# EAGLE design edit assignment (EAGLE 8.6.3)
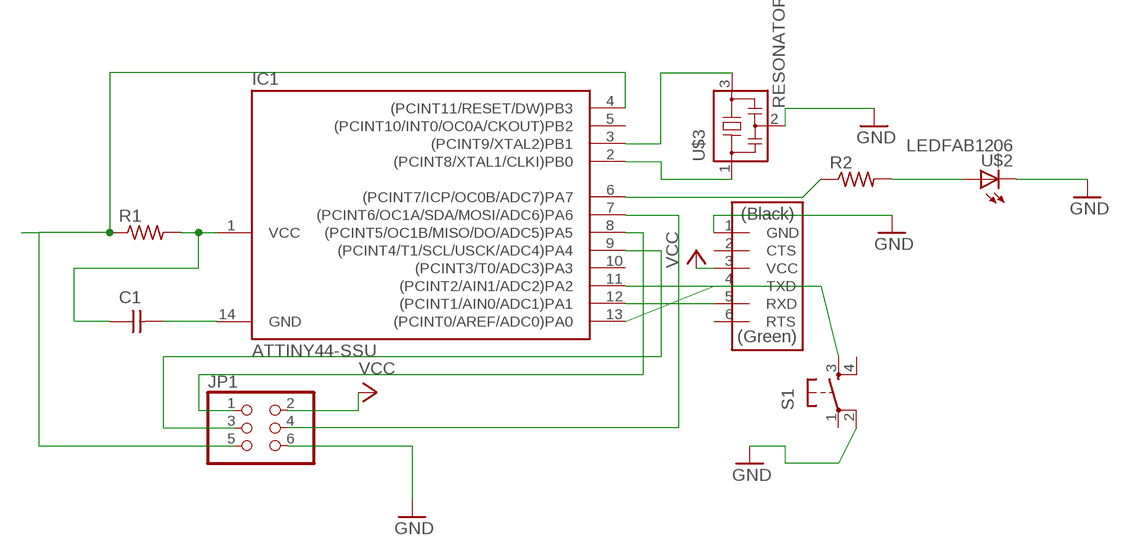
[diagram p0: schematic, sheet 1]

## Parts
C1  CAP-UNPOLARIZEDFAB  [C1206FAB]
IC1  ATTINY44-SSU  [SOIC14]
JP1  PINHD-2X3-SMD  [2X03SMD]
R1  RES-US1206FAB  [R1206FAB]
R2  RES-US1206FAB  [R1206FAB]
S1  6MM_SWITCH6MM_SWITCH  [6MM_SWITCH]
U$1  FTDI-SMD-HEADER  [1X06SMD]
U$2  LEDFAB1206  [LED1206FAB]
U$3  RESONATOR  [EFOBM]

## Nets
GND: JP1.6 S1.2(P1) U$1.1(GND) U$2.2(C) U$3.2
N$1: IC1.4((PCINT11/RESET/DW)PB3) JP1.5 R1.1
N$2: C1.1 IC1.1(VCC) R1.2
N$3: C1.2 IC1.14(GND)
N$4: IC1.13((PCINT0/AREF/ADC0)PA0) U$1.4(TXD)
N$5: IC1.12((PCINT1/AIN0/ADC1)PA1) U$1.5(RXD)
N$6: IC1.8((PCINT5/OC1B/MISO/DO/ADC5)PA5) JP1.1
N$7: IC1.7((PCINT6/OC1A/SDA/MOSI/ADC6)PA6) JP1.4
N$8: IC1.9((PCINT4/T1/SCL/USCK/ADC4)PA4) JP1.3
N$9: IC1.3((PCINT9/XTAL2)PB1) U$3.3
N$10: IC1.2((PCINT8/XTAL1/CLKI)PB0) U$3.1
N$11: IC1.11((PCINT2/AIN1/ADC2)PA2) S1.3(S)
N$12: IC1.6((PCINT7/ICP/OC0B/ADC7)PA7) R2.1
N$13: R2.2 U$2.1(A)
VCC: JP1.2 U$1.3(VCC)
Unconnected: IC1.5((PCINT10/INT0/OC0A/CKOUT)PB2) IC1.10((PCINT3/T0/ADC3)PA3) S1.1(P) S1.4(S1) U$1.2(CTS) U$1.6(RTS)

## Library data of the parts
C1 = fab:CAP-UNPOLARIZED
IC1 = fab:ATTINY44
JP1 = fab:PINHD-2X3-SMD: PIN HEADER
R1 R2 = fab:RES-US: Resistor (US Symbol)
S1 = fab:6MM_SWITCH: OMRON SWITCH
U$1 = fab:FTDI-SMD-HEADER
U$2 = fab:LED: LED
U$3 = fab:RESONATOR

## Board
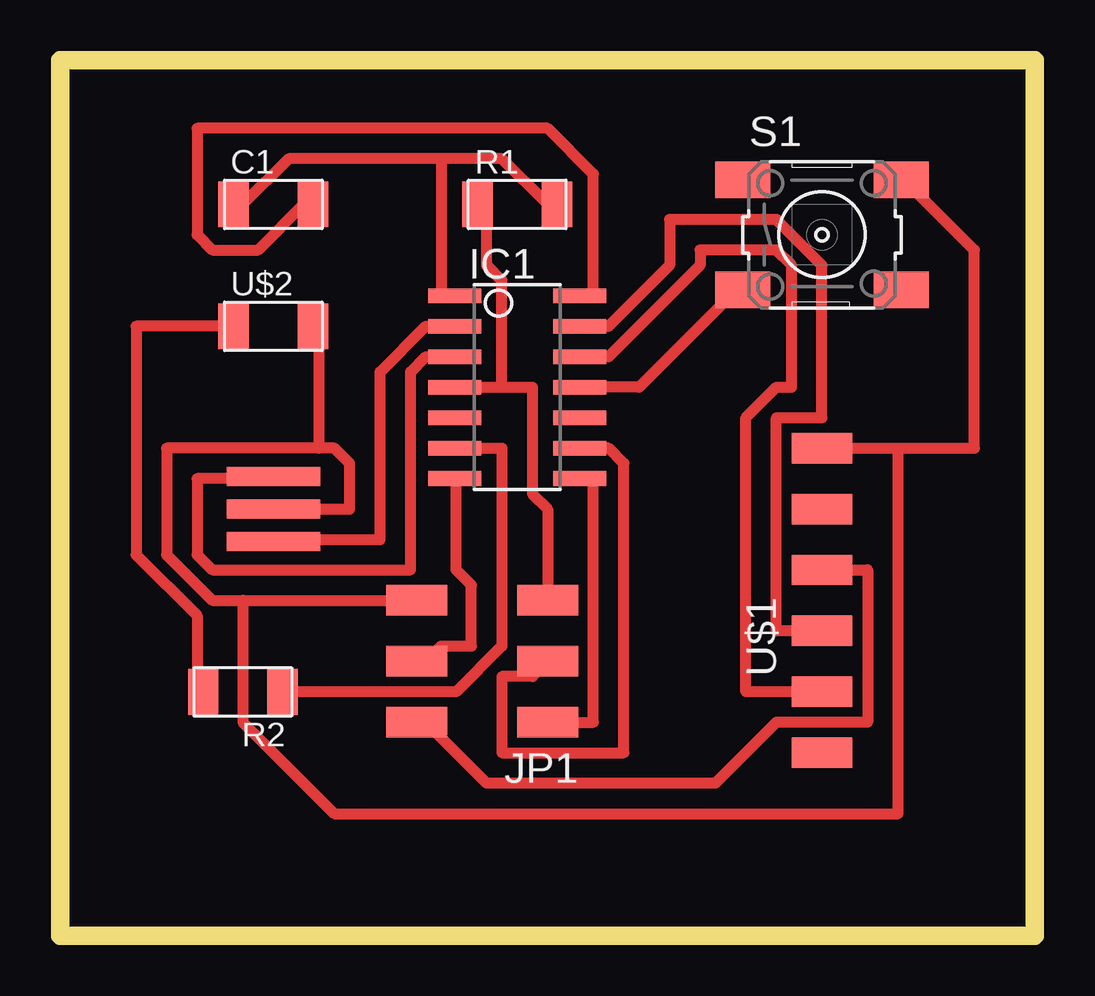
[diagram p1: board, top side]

Size 40.62 x 36.5 mm. Coordinates in mm from the lower left corner, seen from the top.
Outline: 0,0 40.62,0 40.62,36.5 0,36.5 0,0
Copper layers (1*16): Top 0.035mm / dielectric 1.5mm / Bottom 0.035mm
Design rules "default *": minimum track width 18mil, minimum drill 0.35mm, track to track 16mil, track to pad 16mil, pad to pad 16mil, via to via 16mil, smd to smd 16mil, copper to edge 40mil, drill to drill 6mil, minimum pad ring 10mil, minimum via ring 8mil, stop-mask expansion 4mil, vias tented up to drill 0mil, thermal gap 10mil

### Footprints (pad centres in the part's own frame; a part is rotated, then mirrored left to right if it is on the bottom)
C1206FAB = smd 1.27 x 1.905: 1 -1.651,0; 2 1.651,0
SOIC14 = smd 0.61 x 2.21: 1 -3.81,-2.603; 2 -2.54,-2.603; 3 -1.27,-2.603; 4 0,-2.603; 5 1.27,-2.603; 6 2.54,-2.603; 7 3.81,-2.603; 8 3.81,2.603; 9 2.54,2.603; 10 1.27,2.603; 11 0,2.603; 12 -1.27,2.603; 13 -2.54,2.603; 14 -3.81,2.603
2X03SMD = smd 2.54 x 1.27: 1 -2.54,2.54; 2 2.92,2.54; 3 -2.54,0; 4 2.92,0; 5 -2.54,-2.54; 6 2.92,-2.54
R1206FAB = smd 1.27 x 1.905: 1 -1.651,0; 2 1.651,0
6MM_SWITCH = smd 2.286 x 1.524: 1 -3.302,2.286; 2 3.302,2.286; 3 -3.302,-2.286; 4 3.302,-2.286
1X06SMD = smd 2.54 x 1.27: 1 0,6.35; 2 0,3.81; 3 0,1.27; 4 0,-1.27; 5 0,-3.81; 6 0,-6.35
LED1206FAB = smd 1.27 x 1.905: 1 -1.651,0; 2 1.651,0
EFOBM = smd 0.8 x 3.9: 1 -1.35,0; 2 0,0; 3 1.35,0

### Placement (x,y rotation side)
C1  8.89,30.48 0 top
IC1  19.05,22.86 270 top
JP1  17.78,11.43 180 top
R1  19.05,30.48 0 top
R2  7.62,10.16 180 top
S1  31.75,29.21 0 top
U$1  31.75,13.97 0 top
U$2  8.89,25.4 0 top
U$3  8.89,17.78 90 top

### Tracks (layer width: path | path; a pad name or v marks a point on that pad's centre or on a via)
GND
  Top 0.457: U$1.1 34.92,20.32 | 34.92,20.32 38.1,20.32 38.1,28.57 35.56,31.11 S1.2 | 10.79,20.32 10.79,25.4 U$2.2 | 10.79,20.32 11.43,20.32 12.06,19.68 12.06,17.78 U$3.2 | 7.62,13.97 6.35,13.97 4.45,15.88 4.45,20.32 10.79,20.32 | 7.62,13.97 JP1.6 | 34.92,20.32 34.92,5.08 11.43,5.08 7.62,8.89 7.62,13.97
N$1
  Top 0.457: 18.41,22.86 18.41,27.3 17.78,27.94 17.78,30.48 R1.1 | IC1.4 18.41,22.86 | JP1.5 20.32,17.78 19.68,18.41 19.68,22.86 18.41,22.86
N$2
  Top 0.457: 15.88,32.38 18.41,32.38 20.32,30.48 R1.2 | 15.88,32.38 9.52,32.38 7.62,30.48 C1.1 | 15.88,32.38 15.88,26.67 IC1.1
N$3
  Top 0.457: C1.2 10.16,30.48 8.25,28.57 6.35,28.57 5.71,29.21 5.71,33.66 20.32,33.66 22.22,31.75 22.22,26.67 IC1.14
N$4
  Top 0.457: IC1.13 22.86,25.4 25.4,27.94 25.4,29.84 29.84,29.84 31.75,27.94 31.75,21.59 29.84,21.59 29.84,12.7 U$1.4
N$5
  Top 0.457: IC1.12 22.86,24.13 26.67,27.94 26.67,28.57 29.84,28.57 30.48,27.94 30.48,22.86 29.84,22.86 28.57,21.59 28.57,10.16 U$1.5
N$6
  Top 0.457: JP1.1 22.22,8.89 22.22,19.05 IC1.8
N$7
  Top 0.457: IC1.7 16.51,19.05 16.51,15.24 17.14,14.61 17.14,12.06 15.88,12.06 15.24,11.43 JP1.4
N$8
  Top 0.457: IC1.9 22.86,20.32 23.49,19.68 23.49,7.62 18.41,7.62 18.41,10.79 19.68,10.79 JP1.3
N$9
  Top 0.457: IC1.3 15.24,24.13 14.6,23.5 14.6,15.24 6.35,15.24 5.71,15.88 5.71,19.05 8.89,19.05 U$3.3
N$10
  Top 0.457: IC1.2 15.24,25.4 13.33,23.5 13.33,16.51 8.89,16.51 U$3.1
N$11
  Top 0.457: IC1.11 24.13,22.86 27.94,26.67 S1.3
N$12
  Top 0.457: R2.1 16.51,10.16 18.41,12.06 18.41,20.32 IC1.6
N$13
  Top 0.457: U$2.1 3.17,25.4 3.17,15.88 5.71,13.34 5.71,10.16 R2.2
VCC
  Top 0.457: U$1.3 33.65,15.24 33.65,8.89 29.84,8.89 27.3,6.35 17.78,6.35 15.24,8.89 JP1.2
